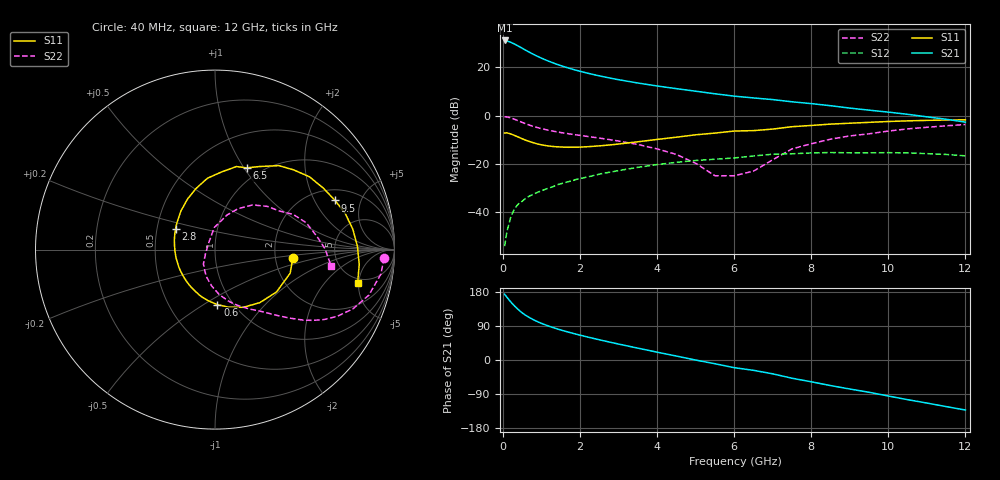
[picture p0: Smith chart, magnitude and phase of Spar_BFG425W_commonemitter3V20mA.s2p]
! Filename: 320bfg425.001
! BFG425W Field C1
! V1=8.504E-001V,V2=3.000E+000V, I1=2.641E-004A, I2=1.998E-002A
# GHz  S  MA  R 50
!  S11  S21  S12  S22
!Freq(GHz)  Mag  Ang  Mag  Ang  Mag  Ang  Mag  Ang
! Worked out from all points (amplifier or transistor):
!   44 points, 40 MHz to 12 GHz, reference 50 ohm
!   highest |S21| = 31.0 dB at 40 MHz (marker M1)
!   |S21| within 3 dB of that: start of sweep to 472.1 MHz
!   unconditionally stable (mu >= 1): 1.389 GHz to end of sweep
!   at 700 MHz: K = 0.74, MSG = 29.6 dB, |S12| = -33.2 dB
!   at 2.4 GHz: K = 1.14, MAG = 18.4 dB, |S12| = -24.6 dB
!   at 12 GHz: K = 1.35, MAG = 3.4 dB, |S12| = -16.7 dB
!   S11 on the Smith chart (normalised r, x): 40 MHz: 2.50, -0.30; 600 MHz: 0.85, -0.57; 2.8 GHz: 0.63, +0.15; 6.5 GHz: 0.86, +1.03; 9.5 GHz: 2.58, +2.97; 12 GHz: 4.37, -4.85
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0.04  0.436 -6.3  35.58 173.5  0.002 65.5  0.942 -2.8
0.1  0.439 -17.4  34.6 165.8  0.004 82.3  0.935 -8.3
0.2  0.416 -34.6  32.57 153.1  0.008 75.9  0.894 -16.5
0.3  0.387 -49.8  29.9 142.2  0.012 71.7  0.836 -23.3
0.4  0.358 -64.0  27.11 132.6  0.015 68.1  0.776 -28.6
0.5  0.33 -76.5  24.48 124.0  0.017 65.2  0.72 -32.8
0.6  0.307 -87.5  22.07 117.1  0.02 63.3  0.67 -36.1
0.7  0.288 -97.3  19.99 111.1  0.022 61.8  0.628 -38.7
0.9  0.258 -114.7  16.63 100.9  0.026 60.0  0.561 -42.7
1  0.248 -122.4  15.29 96.6  0.028 59.3  0.535 -44.4
1.2  0.234 -136.0  13.11 88.9  0.032 58.1  0.493 -47.5
1.6  0.222 -158.9  10.12 76.3  0.041 55.3  0.432 -53.0
2.2  0.227 174.1  7.479 60.5  0.054 50.0  0.369 -61.9
2.8  0.248 152.3  5.892 46.5  0.068 43.3  0.315 -71.7
3.5  0.287 131.5  4.695 31.2  0.085 34.1  0.252 -84.5
4.5  0.357 107.1  3.591 10.4  0.108 19.5  0.157 -108.3
5.5  0.434 85.2  2.812 -9.9  0.125 3.9  0.057 -157.8
6.5  0.488 68.9  2.31 -27.2  0.146 -8.3  0.071 109.8
8.5  0.665 37.6  1.595 -67.5  0.172 -45.3  0.325 50.0
9.5  0.723 22.3  1.291 -85.2  0.17 -62.0  0.419 30.8
10.5  0.776 8.5  1.061 -104.7  0.169 -80.6  0.53 16.4
12  0.816 -13.1  0.73 -132.0  0.147 -110.6  0.652 -7.8
